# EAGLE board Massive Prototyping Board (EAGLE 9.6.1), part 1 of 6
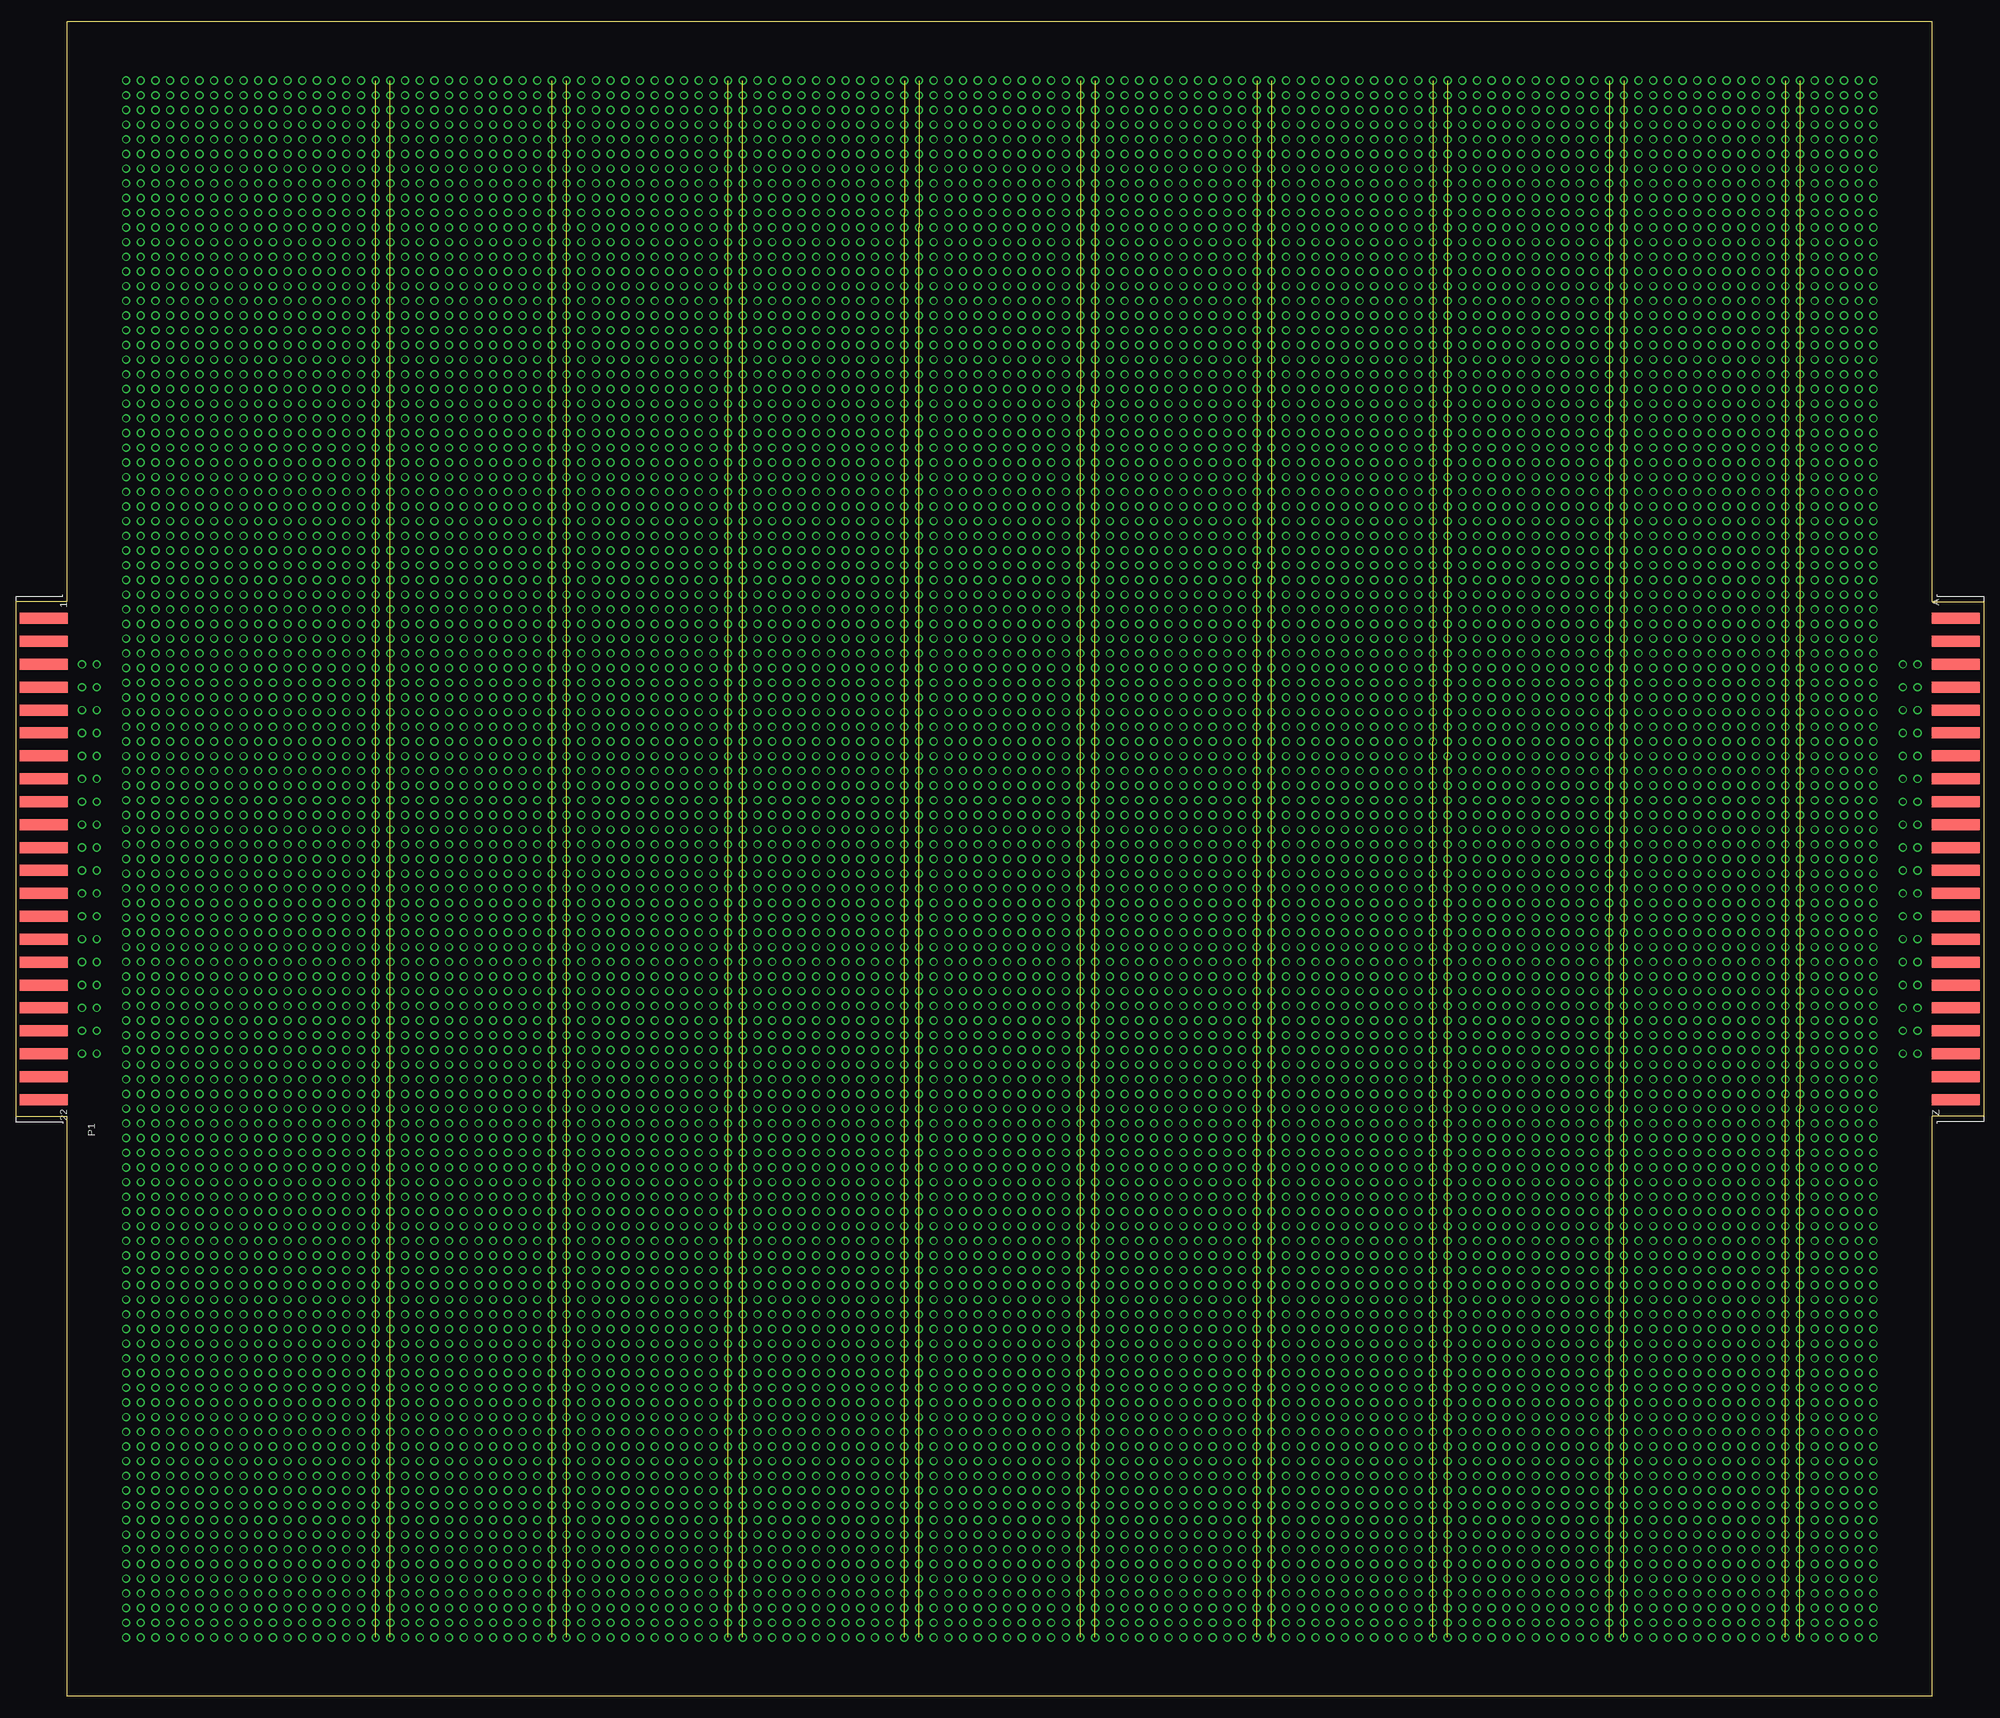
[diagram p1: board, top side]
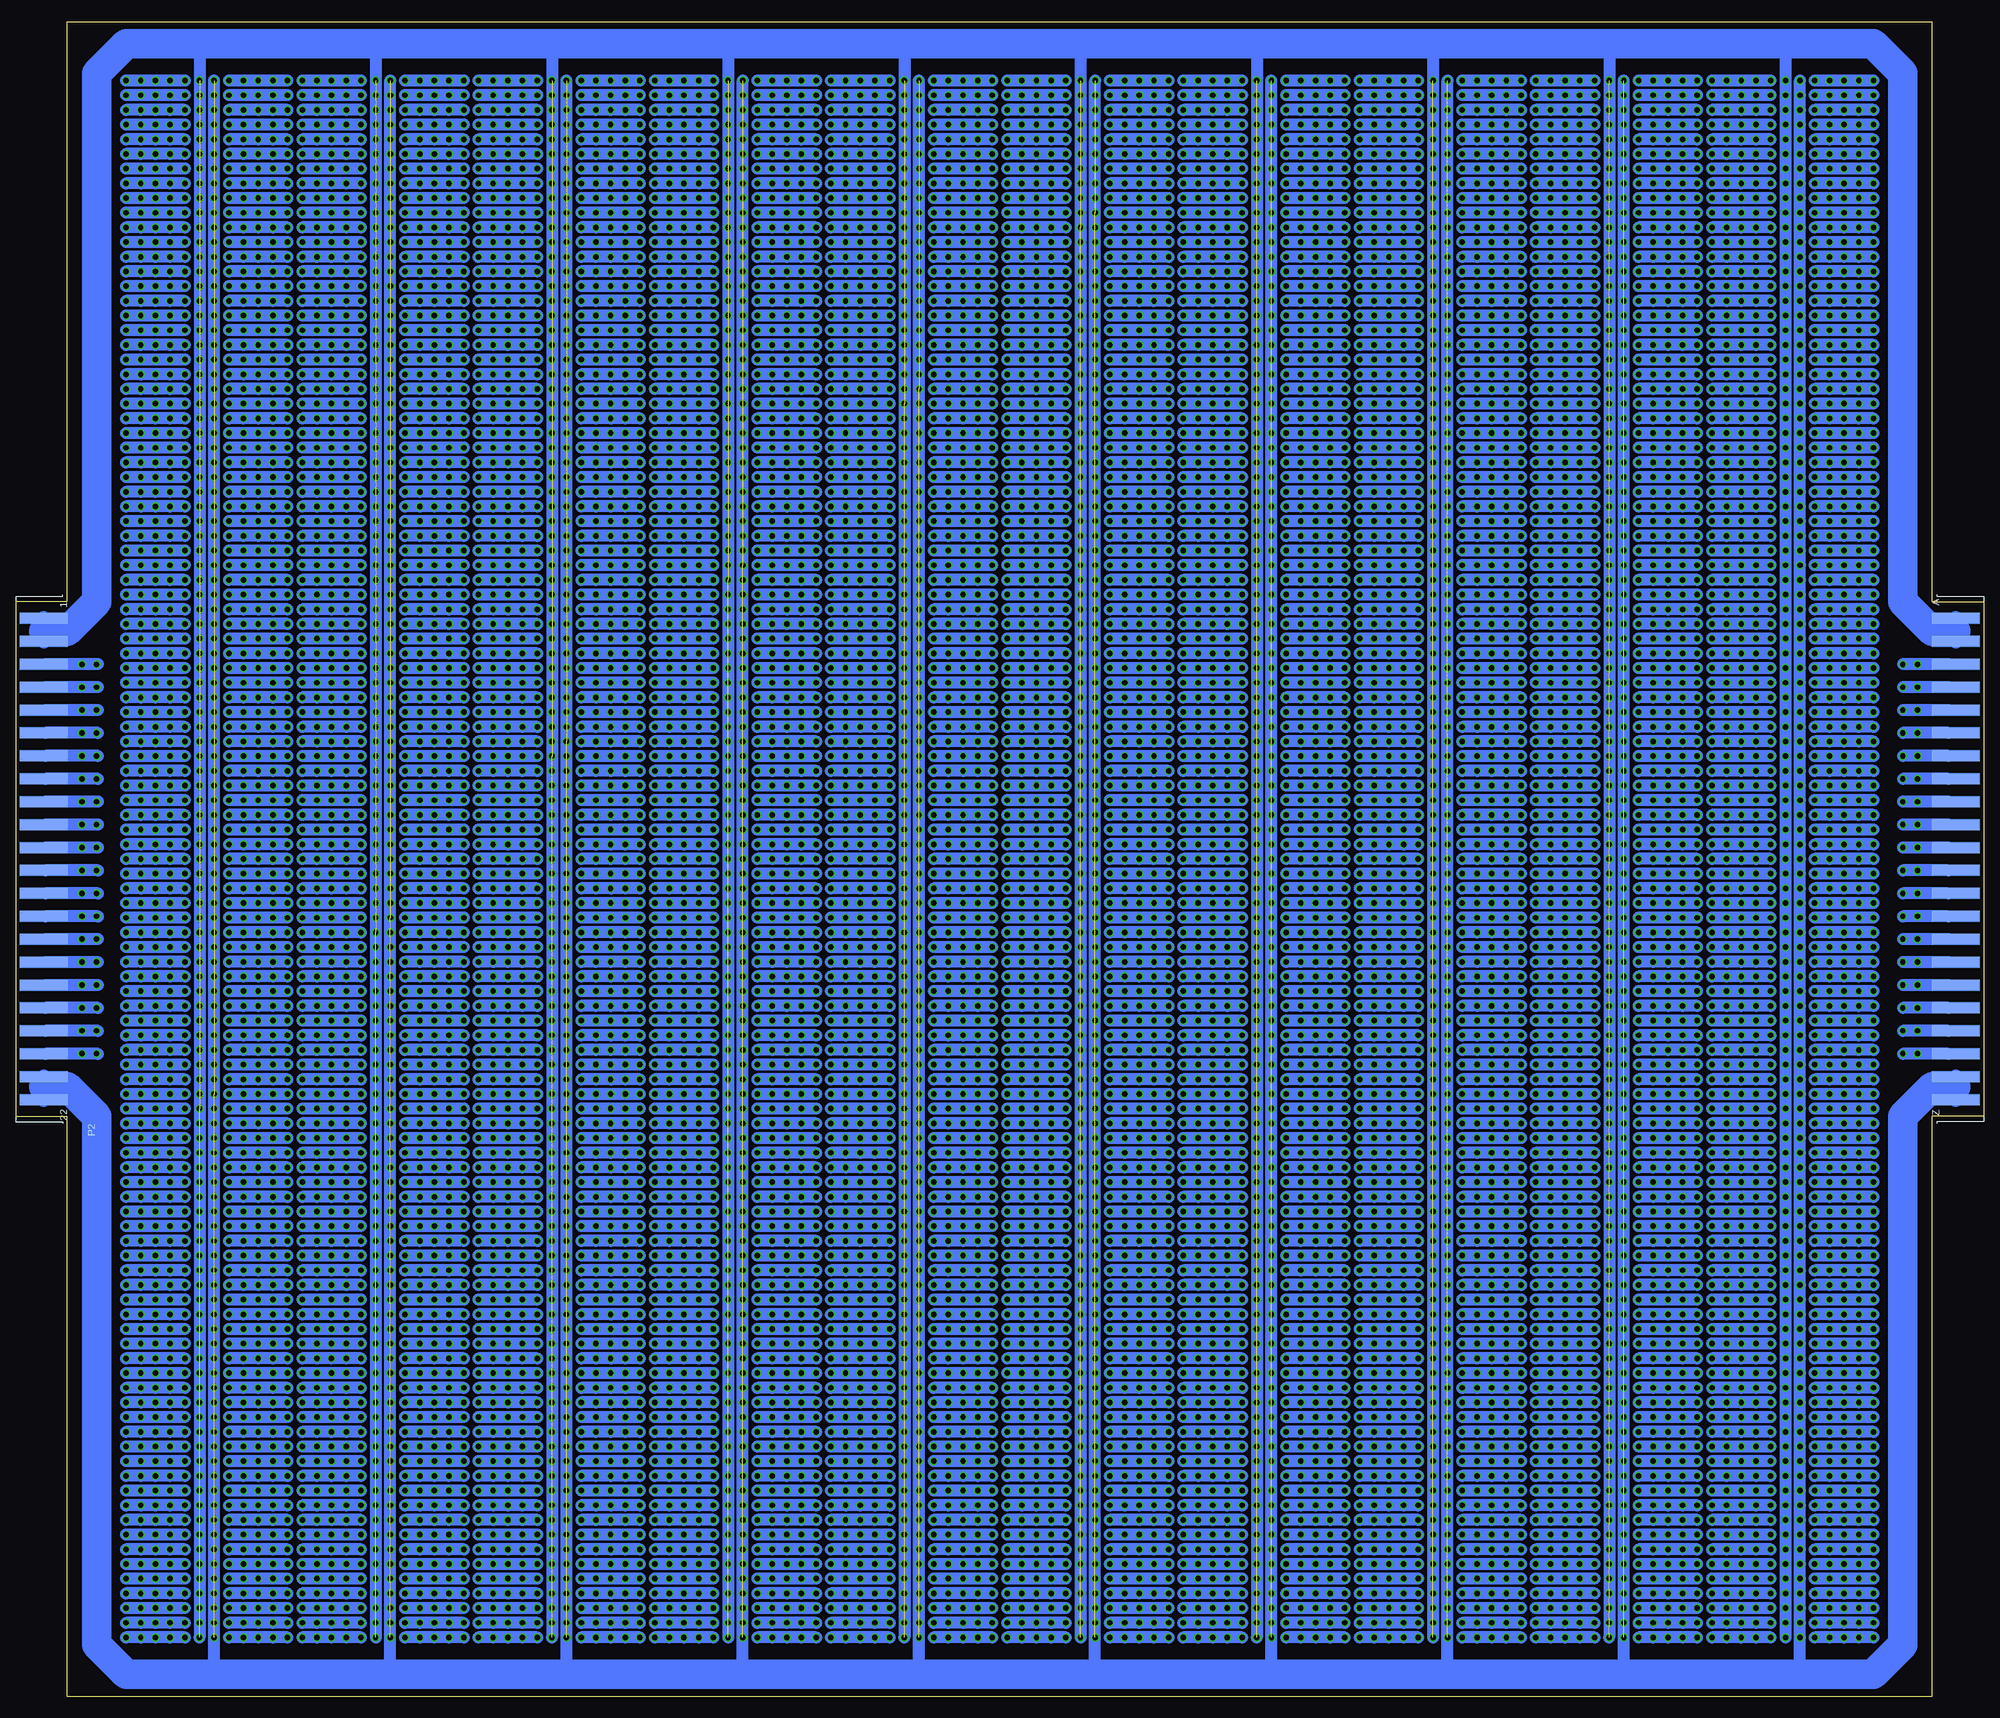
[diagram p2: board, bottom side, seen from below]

Size 340.36 x 289.56 mm. Coordinates in mm from the lower left corner, seen from the top.
Outline: 331.47,0 331.47,100.33 340.36,100.33 340.36,189.23 331.47,189.23 331.47,289.56 8.89,289.56 8.89,189.23 0,189.23 0,100.33 8.89,100.33 8.89,0 331.47,0
Copper layers (1*16): Top 0.035mm / dielectric 1.5mm / Bottom 0.035mm
Design rules "default": minimum track width 6mil, minimum drill 0.35mm, track to track 6mil, track to pad 6mil, pad to pad 6mil, via to via 6mil, smd to smd 6mil, copper to edge 40mil, drill to drill 6mil, minimum pad ring 10mil, minimum via ring 8mil, stop-mask expansion 4mil, vias tented up to drill 0mil, thermal gap 10mil

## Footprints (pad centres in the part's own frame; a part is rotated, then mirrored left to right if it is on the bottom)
44PINEDGE = smd 1.905 x 8.255: 1 -41.605,4.826; 2 -37.643,4.826; 3 -33.68,4.826; 4 -29.718,4.826; 5 -25.756,4.826; 6 -21.793,4.826; 7 -17.831,4.826; 8 -13.868,4.826; 9 -9.906,4.826; 10 -5.944,4.826; 11 -1.981,4.826; 12 1.981,4.826; 13 5.944,4.826; 14 9.906,4.826; 15 13.868,4.826; 16 17.831,4.826; 17 21.793,4.826; 18 25.756,4.826; 19 29.718,4.826; 20 33.68,4.826; 21 37.643,4.826; 22 41.605,4.826 | smd 1.905 x 8.255 bottom: A -41.605,4.826; B -37.643,4.826; C -33.68,4.826; D -29.718,4.826; E -25.756,4.826; F -21.793,4.826; H -17.831,4.826; J -13.868,4.826; K -9.906,4.826; L -5.944,4.826; M -1.981,4.826; N 1.981,4.826; P 5.944,4.826; R 9.906,4.826; S 13.868,4.826; T 17.831,4.826; U 21.793,4.826; V 25.756,4.826; W 29.718,4.826; X 33.68,4.826; Y 37.643,4.826; Z 41.605,4.826

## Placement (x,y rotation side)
P1  44PINEDGE  [44PINEDGE]  0,144.78 270 top
P2  44PINEDGE  [44PINEDGE]  340.36,144.78 270 bottom

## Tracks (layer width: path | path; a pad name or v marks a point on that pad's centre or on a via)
C1
  Bottom 2.032: 6.1,178.46 13.94,178.46
C2
  Bottom 2.032: 326.14,178.46 335.25,178.46
D1
  Bottom 2.032: 6.1,174.5 13.97,174.5
D2
  Bottom 2.032: 326.14,174.5 335.28,174.5
E1
  Bottom 2.032: 6.1,170.54 13.97,170.54
E2
  Bottom 2.032: 326.14,170.54 335.28,170.54
F1
  Bottom 2.032: 6.1,166.57 13.97,166.57
F2
  Bottom 2.032: 326.14,166.57 335.28,166.57
GND  (via drill 0.94)
  Bottom 2.032: 306.07,3.81 306.07,279.4 | 275.59,3.81 275.59,279.4 | 245.11,3.81 245.11,279.4 | 214.63,3.81 214.63,279.4 | 184.15,3.81 184.15,279.4 | 153.67,3.81 153.67,279.4 | 123.19,3.81 123.19,279.4 | 92.71,3.81 92.71,279.4 | 62.23,3.81 62.23,279.4 | 31.75,3.81 v31.75,10.16 v31.75,12.7 v31.75,15.24 v31.75,17.78 v31.75,20.32 v31.75,22.86 v31.75,25.4 v31.75,27.94 v31.75,30.48 v31.75,33.02 v31.75,35.56 v31.75,38.1 v31.75,40.64 v31.75,43.18 v31.75,45.72 v31.75,48.26 v31.75,50.8 v31.75,53.34 v31.75,55.88 v31.75,58.42 v31.75,60.96 v31.75,63.5 v31.75,66.04 v31.75,68.58 v31.75,71.12 v31.75,73.66 v31.75,76.2 v31.75,78.74 v31.75,81.28 v31.75,83.82 v31.75,86.36 v31.75,88.9 v31.75,91.44 v31.75,93.98 v31.75,96.52 v31.75,99.06 v31.75,101.6 v31.75,104.14 v31.75,106.68 v31.75,109.22 v31.75,111.76 v31.75,114.3 v31.75,116.84 v31.75,119.38 v31.75,121.92 v31.75,124.46 v31.75,127 v31.75,129.54 v31.75,132.08 v31.75,134.62 v31.75,137.16 v31.75,139.7 v31.75,142.24 v31.75,144.78 v31.75,147.32 v31.75,149.86 v31.75,152.4 v31.75,154.94 v31.75,157.48 v31.75,160.02 v31.75,162.56 v31.75,165.1 v31.75,167.64 v31.75,170.18 v31.75,172.72 v31.75,175.26 v31.75,177.8 v31.75,180.34 v31.75,182.88 v31.75,185.42 v31.75,187.96 v31.75,190.5 v31.75,193.04 v31.75,195.58 v31.75,198.12 v31.75,200.66 v31.75,203.2 v31.75,205.74 v31.75,208.28 v31.75,210.82 v31.75,213.36 v31.75,215.9 v31.75,218.44 v31.75,220.98 v31.75,223.52 v31.75,226.06 v31.75,228.6 v31.75,231.14 v31.75,233.68 v31.75,236.22 v31.75,238.76 v31.75,241.3 v31.75,243.84 v31.75,246.38 v31.75,248.92 v31.75,251.46 v31.75,254 v31.75,256.54 v31.75,259.08 v31.75,261.62 v31.75,264.16 v31.75,266.7 v31.75,269.24 v31.75,271.78 v31.75,274.32 v31.75,276.86 v31.75,279.4
  Bottom 2.54: P1.Y 4.83,105.41 P1.Z | P2.22 335.53,105.41 P2.21
  Bottom 5.08: 4.83,105.41 8.89,105.41 13.97,100.33 13.97,8.89 19.05,3.81 31.75,3.81 62.23,3.81 92.71,3.81 123.19,3.81 153.67,3.81 184.15,3.81 214.63,3.81 245.11,3.81 275.59,3.81 306.07,3.81 321.31,3.81 326.39,8.89 326.39,100.33 331.47,105.41 335.53,105.41
GND1  (via drill 0.94)  (106 unrouted)
  other vias: 62.23,10.16 62.23,12.7 62.23,15.24 62.23,17.78 62.23,20.32 62.23,22.86 62.23,25.4 62.23,27.94 62.23,30.48 62.23,33.02 62.23,35.56 62.23,38.1 62.23,40.64 62.23,43.18 62.23,45.72 62.23,48.26 62.23,50.8 62.23,53.34 62.23,55.88 62.23,58.42 62.23,63.5 62.23,60.96 62.23,66.04 62.23,68.58 62.23,71.12 62.23,73.66 62.23,76.2 62.23,78.74 62.23,83.82 62.23,81.28 62.23,86.36 62.23,88.9 62.23,91.44 62.23,93.98 62.23,96.52 62.23,99.06 62.23,101.6 62.23,104.14 62.23,106.68 62.23,109.22 62.23,111.76 62.23,114.3 62.23,116.84 62.23,119.38 62.23,121.92 62.23,124.46 62.23,127 62.23,129.54 62.23,132.08 62.23,134.62 62.23,137.16 62.23,139.7 62.23,142.24 62.23,144.78 62.23,147.32 62.23,149.86 62.23,152.4 62.23,154.94 62.23,157.48 62.23,160.02 62.23,162.56 62.23,165.1 62.23,167.64 62.23,170.18 62.23,172.72 62.23,175.26 62.23,177.8 62.23,180.34 62.23,185.42 62.23,182.88 62.23,187.96 62.23,190.5 62.23,193.04 62.23,195.58 62.23,198.12 62.23,200.66 62.23,203.2 62.23,205.74 62.23,208.28 62.23,210.82 62.23,213.36 62.23,215.9 62.23,218.44 62.23,220.98 62.23,223.52 62.23,226.06 62.23,228.6 62.23,231.14 62.23,233.68 62.23,236.22 62.23,238.76 62.23,241.3 62.23,243.84 62.23,246.38 62.23,248.92 62.23,251.46 62.23,254 62.23,256.54 62.23,259.08 62.23,261.62 62.23,264.16 62.23,266.7 62.23,269.24 62.23,271.78 62.23,274.32 62.23,276.86 62.23,279.4
GND2  (via drill 0.94)  (106 unrouted)
  other vias: 92.71,10.16 92.71,12.7 92.71,15.24 92.71,17.78 92.71,20.32 92.71,22.86 92.71,25.4 92.71,27.94 92.71,30.48 92.71,33.02 92.71,35.56 92.71,38.1 92.71,40.64 92.71,43.18 92.71,45.72 92.71,48.26 92.71,50.8 92.71,53.34 92.71,55.88 92.71,58.42 92.71,63.5 92.71,60.96 92.71,66.04 92.71,68.58 92.71,71.12 92.71,73.66 92.71,76.2 92.71,78.74 92.71,83.82 92.71,81.28 92.71,86.36 92.71,88.9 92.71,91.44 92.71,93.98 92.71,96.52 92.71,99.06 92.71,101.6 92.71,104.14 92.71,106.68 92.71,109.22 92.71,111.76 92.71,114.3 92.71,116.84 92.71,119.38 92.71,121.92 92.71,124.46 92.71,127 92.71,129.54 92.71,132.08 92.71,134.62 92.71,137.16 92.71,139.7 92.71,142.24 92.71,144.78 92.71,147.32 92.71,149.86 92.71,152.4 92.71,154.94 92.71,157.48 92.71,160.02 92.71,162.56 92.71,165.1 92.71,167.64 92.71,170.18 92.71,172.72 92.71,175.26 92.71,177.8 92.71,180.34 92.71,185.42 92.71,182.88 92.71,187.96 92.71,190.5 92.71,193.04 92.71,195.58 92.71,198.12 92.71,200.66 92.71,203.2 92.71,205.74 92.71,208.28 92.71,210.82 92.71,213.36 92.71,215.9 92.71,218.44 92.71,220.98 92.71,223.52 92.71,226.06 92.71,228.6 92.71,231.14 92.71,233.68 92.71,236.22 92.71,238.76 92.71,241.3 92.71,243.84 92.71,246.38 92.71,248.92 92.71,251.46 92.71,254 92.71,256.54 92.71,259.08 92.71,261.62 92.71,264.16 92.71,266.7 92.71,269.24 92.71,271.78 92.71,274.32 92.71,276.86 92.71,279.4
GND3  (via drill 0.94)  (106 unrouted)
  other vias: 123.19,10.16 123.19,12.7 123.19,15.24 123.19,17.78 123.19,20.32 123.19,22.86 123.19,25.4 123.19,27.94 123.19,30.48 123.19,33.02 123.19,35.56 123.19,38.1 123.19,40.64 123.19,43.18 123.19,45.72 123.19,48.26 123.19,50.8 123.19,53.34 123.19,55.88 123.19,58.42 123.19,63.5 123.19,60.96 123.19,66.04 123.19,68.58 123.19,71.12 123.19,73.66 123.19,76.2 123.19,78.74 123.19,83.82 123.19,81.28 123.19,86.36 123.19,88.9 123.19,91.44 123.19,93.98 123.19,96.52 123.19,99.06 123.19,101.6 123.19,104.14 123.19,106.68 123.19,109.22 123.19,111.76 123.19,114.3 123.19,116.84 123.19,119.38 123.19,121.92 123.19,124.46 123.19,127 123.19,129.54 123.19,132.08 123.19,134.62 123.19,137.16 123.19,139.7 123.19,142.24 123.19,144.78 123.19,147.32 123.19,149.86 123.19,152.4 123.19,154.94 123.19,157.48 123.19,160.02 123.19,162.56 123.19,165.1 123.19,167.64 123.19,170.18 123.19,172.72 123.19,175.26 123.19,177.8 123.19,180.34 123.19,185.42 123.19,182.88 123.19,187.96 123.19,190.5 123.19,193.04 123.19,195.58 123.19,198.12 123.19,200.66 123.19,203.2 123.19,205.74 123.19,208.28 123.19,210.82 123.19,213.36 123.19,215.9 123.19,218.44 123.19,220.98 123.19,223.52 123.19,226.06 123.19,228.6 123.19,231.14 123.19,233.68 123.19,236.22 123.19,238.76 123.19,241.3 123.19,243.84 123.19,246.38 123.19,248.92 123.19,251.46 123.19,254 123.19,256.54 123.19,259.08 123.19,261.62 123.19,264.16 123.19,266.7 123.19,269.24 123.19,271.78 123.19,274.32 123.19,276.86 123.19,279.4
GND4  (via drill 0.94)  (106 unrouted)
  other vias: 153.67,10.16 153.67,12.7 153.67,15.24 153.67,17.78 153.67,20.32 153.67,22.86 153.67,25.4 153.67,27.94 153.67,30.48 153.67,33.02 153.67,35.56 153.67,38.1 153.67,40.64 153.67,43.18 153.67,45.72 153.67,48.26 153.67,50.8 153.67,53.34 153.67,55.88 153.67,58.42 153.67,63.5 153.67,60.96 153.67,66.04 153.67,68.58 153.67,71.12 153.67,73.66 153.67,76.2 153.67,78.74 153.67,83.82 153.67,81.28 153.67,86.36 153.67,88.9 153.67,91.44 153.67,93.98 153.67,96.52 153.67,99.06 153.67,101.6 153.67,104.14 153.67,106.68 153.67,109.22 153.67,111.76 153.67,114.3 153.67,116.84 153.67,119.38 153.67,121.92 153.67,124.46 153.67,127 153.67,129.54 153.67,132.08 153.67,134.62 153.67,137.16 153.67,139.7 153.67,142.24 153.67,144.78 153.67,147.32 153.67,149.86 153.67,152.4 153.67,154.94 153.67,157.48 153.67,160.02 153.67,162.56 153.67,165.1 153.67,167.64 153.67,170.18 153.67,172.72 153.67,175.26 153.67,177.8 153.67,180.34 153.67,185.42 153.67,182.88 153.67,187.96 153.67,190.5 153.67,193.04 153.67,195.58 153.67,198.12 153.67,200.66 153.67,203.2 153.67,205.74 153.67,208.28 153.67,210.82 153.67,213.36 153.67,215.9 153.67,218.44 153.67,220.98 153.67,223.52 153.67,226.06 153.67,228.6 153.67,231.14 153.67,233.68 153.67,236.22 153.67,238.76 153.67,241.3 153.67,243.84 153.67,246.38 153.67,248.92 153.67,251.46 153.67,254 153.67,256.54 153.67,259.08 153.67,261.62 153.67,264.16 153.67,266.7 153.67,269.24 153.67,271.78 153.67,274.32 153.67,276.86 153.67,279.4
GND5  (via drill 0.94)  (106 unrouted)
  other vias: 184.15,10.16 184.15,12.7 184.15,15.24 184.15,17.78 184.15,20.32 184.15,22.86 184.15,25.4 184.15,27.94 184.15,30.48 184.15,33.02 184.15,35.56 184.15,38.1 184.15,40.64 184.15,43.18 184.15,45.72 184.15,48.26 184.15,50.8 184.15,53.34 184.15,55.88 184.15,58.42 184.15,63.5 184.15,60.96 184.15,66.04 184.15,68.58 184.15,71.12 184.15,73.66 184.15,76.2 184.15,78.74 184.15,83.82 184.15,81.28 184.15,86.36 184.15,88.9 184.15,91.44 184.15,93.98 184.15,96.52 184.15,99.06 184.15,101.6 184.15,104.14 184.15,106.68 184.15,109.22 184.15,111.76 184.15,114.3 184.15,116.84 184.15,119.38 184.15,121.92 184.15,124.46 184.15,127 184.15,129.54 184.15,132.08 184.15,134.62 184.15,137.16 184.15,139.7 184.15,142.24 184.15,144.78 184.15,147.32 184.15,149.86 184.15,152.4 184.15,154.94 184.15,157.48 184.15,160.02 184.15,162.56 184.15,165.1 184.15,167.64 184.15,170.18 184.15,172.72 184.15,175.26 184.15,177.8 184.15,180.34 184.15,185.42 184.15,182.88 184.15,187.96 184.15,190.5 184.15,193.04 184.15,195.58 184.15,198.12 184.15,200.66 184.15,203.2 184.15,205.74 184.15,208.28 184.15,210.82 184.15,213.36 184.15,215.9 184.15,218.44 184.15,220.98 184.15,223.52 184.15,226.06 184.15,228.6 184.15,231.14 184.15,233.68 184.15,236.22 184.15,238.76 184.15,241.3 184.15,243.84 184.15,246.38 184.15,248.92 184.15,251.46 184.15,254 184.15,256.54 184.15,259.08 184.15,261.62 184.15,264.16 184.15,266.7 184.15,269.24 184.15,271.78 184.15,274.32 184.15,276.86 184.15,279.4
GND6  (via drill 0.94)  (106 unrouted)
  other vias: 214.63,10.16 214.63,12.7 214.63,15.24 214.63,17.78 214.63,20.32 214.63,22.86 214.63,25.4 214.63,27.94 214.63,30.48 214.63,33.02 214.63,35.56 214.63,38.1 214.63,40.64 214.63,43.18 214.63,45.72 214.63,48.26 214.63,50.8 214.63,53.34 214.63,55.88 214.63,58.42 214.63,63.5 214.63,60.96 214.63,66.04 214.63,68.58 214.63,71.12 214.63,73.66 214.63,76.2 214.63,78.74 214.63,83.82 214.63,81.28 214.63,86.36 214.63,88.9 214.63,91.44 214.63,93.98 214.63,96.52 214.63,99.06 214.63,101.6 214.63,104.14 214.63,106.68 214.63,109.22 214.63,111.76 214.63,114.3 214.63,116.84 214.63,119.38 214.63,121.92 214.63,124.46 214.63,127 214.63,129.54 214.63,132.08 214.63,134.62 214.63,137.16 214.63,139.7 214.63,142.24 214.63,144.78 214.63,147.32 214.63,149.86 214.63,152.4 214.63,154.94 214.63,157.48 214.63,160.02 214.63,162.56 214.63,165.1 214.63,167.64 214.63,170.18 214.63,172.72 214.63,175.26 214.63,177.8 214.63,180.34 214.63,185.42 214.63,182.88 214.63,187.96 214.63,190.5 214.63,193.04 214.63,195.58 214.63,198.12 214.63,200.66 214.63,203.2 214.63,205.74 214.63,208.28 214.63,210.82 214.63,213.36 214.63,215.9 214.63,218.44 214.63,220.98 214.63,223.52 214.63,226.06 214.63,228.6 214.63,231.14 214.63,233.68 214.63,236.22 214.63,238.76 214.63,241.3 214.63,243.84 214.63,246.38 214.63,248.92 214.63,251.46 214.63,254 214.63,256.54 214.63,259.08 214.63,261.62 214.63,264.16 214.63,266.7 214.63,269.24 214.63,271.78 214.63,274.32 214.63,276.86 214.63,279.4
GND7  (via drill 0.94)  (106 unrouted)
  other vias: 245.11,10.16 245.11,12.7 245.11,15.24 245.11,17.78 245.11,20.32 245.11,22.86 245.11,25.4 245.11,27.94 245.11,30.48 245.11,33.02 245.11,35.56 245.11,38.1 245.11,40.64 245.11,43.18 245.11,45.72 245.11,48.26 245.11,50.8 245.11,53.34 245.11,55.88 245.11,58.42 245.11,63.5 245.11,60.96 245.11,66.04 245.11,68.58 245.11,71.12 245.11,73.66 245.11,76.2 245.11,78.74 245.11,83.82 245.11,81.28 245.11,86.36 245.11,88.9 245.11,91.44 245.11,93.98 245.11,96.52 245.11,99.06 245.11,101.6 245.11,104.14 245.11,106.68 245.11,109.22 245.11,111.76 245.11,114.3 245.11,116.84 245.11,119.38 245.11,121.92 245.11,124.46 245.11,127 245.11,129.54 245.11,132.08 245.11,134.62 245.11,137.16 245.11,139.7 245.11,142.24 245.11,144.78 245.11,147.32 245.11,149.86 245.11,152.4 245.11,154.94 245.11,157.48 245.11,160.02 245.11,162.56 245.11,165.1 245.11,167.64 245.11,170.18 245.11,172.72 245.11,175.26 245.11,177.8 245.11,180.34 245.11,185.42 245.11,182.88 245.11,187.96 245.11,190.5 245.11,193.04 245.11,195.58 245.11,198.12 245.11,200.66 245.11,203.2 245.11,205.74 245.11,208.28 245.11,210.82 245.11,213.36 245.11,215.9 245.11,218.44 245.11,220.98 245.11,223.52 245.11,226.06 245.11,228.6 245.11,231.14 245.11,233.68 245.11,236.22 245.11,238.76 245.11,241.3 245.11,243.84 245.11,246.38 245.11,248.92 245.11,251.46 245.11,254 245.11,256.54 245.11,259.08 245.11,261.62 245.11,264.16 245.11,266.7 245.11,269.24 245.11,271.78 245.11,274.32 245.11,276.86 245.11,279.4
GND8  (via drill 0.94)  (106 unrouted)
  other vias: 275.59,10.16 275.59,12.7 275.59,15.24 275.59,17.78 275.59,20.32 275.59,22.86 275.59,25.4 275.59,27.94 275.59,30.48 275.59,33.02 275.59,35.56 275.59,38.1 275.59,40.64 275.59,43.18 275.59,45.72 275.59,48.26 275.59,50.8 275.59,53.34 275.59,55.88 275.59,58.42 275.59,63.5 275.59,60.96 275.59,66.04 275.59,68.58 275.59,71.12 275.59,73.66 275.59,76.2 275.59,78.74 275.59,83.82 275.59,81.28 275.59,86.36 275.59,88.9 275.59,91.44 275.59,93.98 275.59,96.52 275.59,99.06 275.59,101.6 275.59,104.14 275.59,106.68 275.59,109.22 275.59,111.76 275.59,114.3 275.59,116.84 275.59,119.38 275.59,121.92 275.59,124.46 275.59,127 275.59,129.54 275.59,132.08 275.59,134.62 275.59,137.16 275.59,139.7 275.59,142.24 275.59,144.78 275.59,147.32 275.59,149.86 275.59,152.4 275.59,154.94 275.59,157.48 275.59,160.02 275.59,162.56 275.59,165.1 275.59,167.64 275.59,170.18 275.59,172.72 275.59,175.26 275.59,177.8 275.59,180.34 275.59,185.42 275.59,182.88 275.59,187.96 275.59,190.5 275.59,193.04 275.59,195.58 275.59,198.12 275.59,200.66 275.59,203.2 275.59,205.74 275.59,208.28 275.59,210.82 275.59,213.36 275.59,215.9 275.59,218.44 275.59,220.98 275.59,223.52 275.59,226.06 275.59,228.6 275.59,231.14 275.59,233.68 275.59,236.22 275.59,238.76 275.59,241.3 275.59,243.84 275.59,246.38 275.59,248.92 275.59,251.46 275.59,254 275.59,256.54 275.59,259.08 275.59,261.62 275.59,264.16 275.59,266.7 275.59,269.24 275.59,271.78 275.59,274.32 275.59,276.86 275.59,279.4
GND9  (via drill 0.94)  (106 unrouted)
  other vias: 306.07,10.16 306.07,12.7 306.07,15.24 306.07,17.78 306.07,20.32 306.07,22.86 306.07,25.4 306.07,27.94 306.07,30.48 306.07,33.02 306.07,35.56 306.07,38.1 306.07,40.64 306.07,43.18 306.07,45.72 306.07,48.26 306.07,50.8 306.07,53.34 306.07,55.88 306.07,58.42 306.07,63.5 306.07,60.96 306.07,66.04 306.07,68.58 306.07,71.12 306.07,73.66 306.07,76.2 306.07,78.74 306.07,83.82 306.07,81.28 306.07,86.36 306.07,88.9 306.07,91.44 306.07,93.98 306.07,96.52 306.07,99.06 306.07,101.6 306.07,104.14 306.07,106.68 306.07,109.22 306.07,111.76 306.07,114.3 306.07,116.84 306.07,119.38 306.07,121.92 306.07,124.46 306.07,127 306.07,129.54 306.07,132.08 306.07,134.62 306.07,137.16 306.07,139.7 306.07,142.24 306.07,144.78 306.07,147.32 306.07,149.86 306.07,152.4 306.07,154.94 306.07,157.48 306.07,160.02 306.07,162.56 306.07,165.1 306.07,167.64 306.07,170.18 306.07,172.72 306.07,175.26 306.07,177.8 306.07,180.34 306.07,185.42 306.07,182.88 306.07,187.96 306.07,190.5 306.07,193.04 306.07,195.58 306.07,198.12 306.07,200.66 306.07,203.2 306.07,205.74 306.07,208.28 306.07,210.82 306.07,213.36 306.07,215.9 306.07,218.44 306.07,220.98 306.07,223.52 306.07,226.06 306.07,228.6 306.07,231.14 306.07,233.68 306.07,236.22 306.07,238.76 306.07,241.3 306.07,243.84 306.07,246.38 306.07,248.92 306.07,251.46 306.07,254 306.07,256.54 306.07,259.08 306.07,261.62 306.07,264.16 306.07,266.7 306.07,269.24 306.07,271.78 306.07,274.32 306.07,276.86 306.07,279.4
H1
  Bottom 2.032: 6.1,162.61 13.97,162.61
H2
  Bottom 2.032: 326.14,162.61 335.28,162.61
J1
  Bottom 2.032: 6.1,158.65 13.97,158.65
J2
  Bottom 2.032: 326.14,158.65 335.28,158.65
K1
  Bottom 2.032: 6.1,154.69 13.97,154.69
K2
  Bottom 2.032: 326.14,154.69 335.28,154.69
L1
  Bottom 2.032: 6.1,150.72 13.97,150.72
L2
  Bottom 2.032: 326.14,150.72 335.28,150.72
M1
  Bottom 2.032: 6.1,146.76 13.97,146.76
M2
  Bottom 2.032: 326.14,146.76 335.28,146.76
N1
  Bottom 2.032: 6.1,142.8 13.97,142.8
N2
  Bottom 2.032: 326.14,142.8 335.28,142.8
N$1  (via drill 0.94)
  Bottom 2.032: v36.83,12.7 v39.37,12.7 v41.91,12.7 v44.45,12.7 v46.99,12.7
N$2  (via drill 0.94)
  Bottom 2.032: v36.83,15.24 v39.37,15.24 v41.91,15.24 v44.45,15.24 v46.99,15.24
N$3  (via drill 0.94)
  Bottom 2.032: v36.83,17.78 v39.37,17.78 v41.91,17.78 v44.45,17.78 v46.99,17.78
N$4  (via drill 0.94)
  Bottom 2.032: v36.83,20.32 v39.37,20.32 v41.91,20.32 v44.45,20.32 v46.99,20.32
N$5  (via drill 0.94)
  Bottom 2.032: v36.83,22.86 v39.37,22.86 v41.91,22.86 v44.45,22.86 v46.99,22.86
N$6  (via drill 0.94)
  Bottom 2.032: v36.83,25.4 v39.37,25.4 v41.91,25.4 v44.45,25.4 v46.99,25.4
N$7  (via drill 0.94)
  Bottom 2.032: v36.83,27.94 v39.37,27.94 v41.91,27.94 v44.45,27.94 v46.99,27.94
N$8  (via drill 0.94)
  Bottom 2.032: v36.83,30.48 v39.37,30.48 v41.91,30.48 v44.45,30.48 v46.99,30.48
N$9  (via drill 0.94)
  Bottom 2.032: v36.83,33.02 v39.37,33.02 v41.91,33.02 v44.45,33.02 v46.99,33.02
N$10  (via drill 0.94)
  Bottom 2.032: v36.83,35.56 v39.37,35.56 v41.91,35.56 v44.45,35.56 v46.99,35.56
N$11  (via drill 0.94)
  Bottom 2.032: v36.83,38.1 v39.37,38.1 v41.91,38.1 v44.45,38.1 v46.99,38.1
N$12  (via drill 0.94)
  Bottom 2.032: v36.83,40.64 v39.37,40.64 v41.91,40.64 v44.45,40.64 v46.99,40.64
N$13  (via drill 0.94)
  Bottom 2.032: v36.83,43.18 v39.37,43.18 v41.91,43.18 v44.45,43.18 v46.99,43.18
N$14  (via drill 0.94)
  Bottom 2.032: v36.83,45.72 v39.37,45.72 v41.91,45.72 v44.45,45.72 v46.99,45.72
N$15  (via drill 0.94)
  Bottom 2.032: v36.83,48.26 v39.37,48.26 v41.91,48.26 v44.45,48.26 v46.99,48.26
N$16  (via drill 0.94)
  Bottom 2.032: v36.83,50.8 v39.37,50.8 v41.91,50.8 v44.45,50.8 v46.99,50.8
N$17  (via drill 0.94)
  Bottom 2.032: v36.83,53.34 v39.37,53.34 v41.91,53.34 v44.45,53.34 v46.99,53.34
N$18  (via drill 0.94)
  Bottom 2.032: v36.83,55.88 v39.37,55.88 v41.91,55.88 v44.45,55.88 v46.99,55.88
N$19  (via drill 0.94)
  Bottom 2.032: v36.83,58.42 v39.37,58.42 v41.91,58.42 v44.45,58.42 v46.99,58.42
N$20  (via drill 0.94)
  Bottom 2.032: v36.83,60.96 v39.37,60.96 v41.91,60.96 v44.45,60.96 v46.99,60.96
N$21  (via drill 0.94)
  Bottom 2.032: v36.83,63.5 v39.37,63.5 v41.91,63.5 v44.45,63.5 v46.99,63.5
N$22  (via drill 0.94)
  Bottom 2.032: v36.83,66.04 v39.37,66.04 v41.91,66.04 v44.45,66.04 v46.99,66.04
N$23  (via drill 0.94)
  Bottom 2.032: v36.83,68.58 v39.37,68.58 v41.91,68.58 v44.45,68.58 v46.99,68.58
N$24  (via drill 0.94)
  Bottom 2.032: v36.83,71.12 v39.37,71.12 v41.91,71.12 v44.45,71.12 v46.99,71.12
N$25  (via drill 0.94)
  Bottom 2.032: v36.83,73.66 v39.37,73.66 v41.91,73.66 v44.45,73.66 v46.99,73.66
N$26  (via drill 0.94)
  Bottom 2.032: v36.83,76.2 v39.37,76.2 v41.91,76.2 v44.45,76.2 v46.99,76.2
N$27  (via drill 0.94)
  Bottom 2.032: v36.83,78.74 v39.37,78.74 v41.91,78.74 v44.45,78.74 v46.99,78.74
N$28  (via drill 0.94)
  Bottom 2.032: v36.83,81.28 v39.37,81.28 v41.91,81.28 v44.45,81.28 v46.99,81.28
N$29  (via drill 0.94)
  Bottom 2.032: v36.83,83.82 v39.37,83.82 v41.91,83.82 v44.45,83.82 v46.99,83.82
N$30  (via drill 0.94)
  Bottom 2.032: v36.83,86.36 v39.37,86.36 v41.91,86.36 v44.45,86.36 v46.99,86.36
N$31  (via drill 0.94)
  Bottom 2.032: v36.83,88.9 v39.37,88.9 v41.91,88.9 v44.45,88.9 v46.99,88.9
N$32  (via drill 0.94)
  Bottom 2.032: v36.83,91.44 v39.37,91.44 v41.91,91.44 v44.45,91.44 v46.99,91.44
N$33  (via drill 0.94)
  Bottom 2.032: v36.83,93.98 v39.37,93.98 v41.91,93.98 v44.45,93.98 v46.99,93.98
N$34  (via drill 0.94)
  Bottom 2.032: v36.83,96.52 v39.37,96.52 v41.91,96.52 v44.45,96.52 v46.99,96.52
N$35  (via drill 0.94)
  Bottom 2.032: v36.83,99.06 v39.37,99.06 v41.91,99.06 v44.45,99.06 v46.99,99.06
N$36  (via drill 0.94)
  Bottom 2.032: v36.83,101.6 v39.37,101.6 v41.91,101.6 v44.45,101.6 v46.99,101.6
N$37  (via drill 0.94)
  Bottom 2.032: v36.83,104.14 v39.37,104.14 v41.91,104.14 v44.45,104.14 v46.99,104.14
N$38  (via drill 0.94)
  Bottom 2.032: v36.83,106.68 v39.37,106.68 v41.91,106.68 v44.45,106.68 v46.99,106.68
N$39  (via drill 0.94)
  Bottom 2.032: v36.83,109.22 v39.37,109.22 v41.91,109.22 v44.45,109.22 v46.99,109.22
N$40  (via drill 0.94)
  Bottom 2.032: v36.83,111.76 v39.37,111.76 v41.91,111.76 v44.45,111.76 v46.99,111.76
N$41  (via drill 0.94)
  Bottom 2.032: v36.83,114.3 v39.37,114.3 v41.91,114.3 v44.45,114.3 v46.99,114.3
N$42  (via drill 0.94)
  Bottom 2.032: v36.83,116.84 v39.37,116.84 v41.91,116.84 v44.45,116.84 v46.99,116.84
N$43  (via drill 0.94)
  Bottom 2.032: v36.83,119.38 v39.37,119.38 v41.91,119.38 v44.45,119.38 v46.99,119.38
N$44  (via drill 0.94)
  Bottom 2.032: v36.83,121.92 v39.37,121.92 v41.91,121.92 v44.45,121.92 v46.99,121.92
N$45  (via drill 0.94)
  Bottom 2.032: v36.83,124.46 v39.37,124.46 v41.91,124.46 v44.45,124.46 v46.99,124.46
N$46  (via drill 0.94)
  Bottom 2.032: v36.83,127 v39.37,127 v41.91,127 v44.45,127 v46.99,127
N$47  (via drill 0.94)
  Bottom 2.032: v36.83,129.54 v39.37,129.54 v41.91,129.54 v44.45,129.54 v46.99,129.54
N$48  (via drill 0.94)
  Bottom 2.032: v36.83,132.08 v39.37,132.08 v41.91,132.08 v44.45,132.08 v46.99,132.08
N$49  (via drill 0.94)
  Bottom 2.032: v36.83,134.62 v39.37,134.62 v41.91,134.62 v44.45,134.62 v46.99,134.62
N$50  (via drill 0.94)
  Bottom 2.032: v36.83,137.16 v39.37,137.16 v41.91,137.16 v44.45,137.16 v46.99,137.16
N$51  (via drill 0.94)
  Bottom 2.032: v36.83,139.7 v39.37,139.7 v41.91,139.7 v44.45,139.7 v46.99,139.7
N$52  (via drill 0.94)
  Bottom 2.032: v36.83,142.24 v39.37,142.24 v41.91,142.24 v44.45,142.24 v46.99,142.24
N$53  (via drill 0.94)
  Bottom 2.032: v36.83,144.78 v39.37,144.78 v41.91,144.78 v44.45,144.78 v46.99,144.78
N$54  (via drill 0.94)
  Bottom 2.032: v36.83,147.32 v39.37,147.32 v41.91,147.32 v44.45,147.32 v46.99,147.32
N$55  (via drill 0.94)
  Bottom 2.032: v36.83,149.86 v39.37,149.86 v41.91,149.86 v44.45,149.86 v46.99,149.86
N$56  (via drill 0.94)
  Bottom 2.032: v36.83,152.4 v39.37,152.4 v41.91,152.4 v44.45,152.4 v46.99,152.4
N$57  (via drill 0.94)
  Bottom 2.032: v36.83,154.94 v39.37,154.94 v41.91,154.94 v44.45,154.94 v46.99,154.94
N$58  (via drill 0.94)
  Bottom 2.032: v36.83,157.48 v39.37,157.48 v41.91,157.48 v44.45,157.48 v46.99,157.48
N$59  (via drill 0.94)
  Bottom 2.032: v36.83,160.02 v39.37,160.02 v41.91,160.02 v44.45,160.02 v46.99,160.02
N$60  (via drill 0.94)
  Bottom 2.032: v36.83,162.56 v39.37,162.56 v41.91,162.56 v44.45,162.56 v46.99,162.56
N$61  (via drill 0.94)
  Bottom 2.032: v36.83,165.1 v39.37,165.1 v41.91,165.1 v44.45,165.1 v46.99,165.1
N$62  (via drill 0.94)
  Bottom 2.032: v36.83,167.64 v39.37,167.64 v41.91,167.64 v44.45,167.64 v46.99,167.64
N$63  (via drill 0.94)
  Bottom 2.032: v36.83,170.18 v39.37,170.18 v41.91,170.18 v44.45,170.18 v46.99,170.18
N$64  (via drill 0.94)
  Bottom 2.032: v36.83,172.72 v39.37,172.72 v41.91,172.72 v44.45,172.72 v46.99,172.72
N$65  (via drill 0.94)
  Bottom 2.032: v36.83,175.26 v39.37,175.26 v41.91,175.26 v44.45,175.26 v46.99,175.26
N$66  (via drill 0.94)
  Bottom 2.032: v36.83,177.8 v39.37,177.8 v41.91,177.8 v44.45,177.8 v46.99,177.8
N$67  (via drill 0.94)
  Bottom 2.032: v36.83,180.34 v39.37,180.34 v41.91,180.34 v44.45,180.34 v46.99,180.34
N$68  (via drill 0.94)
  Bottom 2.032: v36.83,182.88 v39.37,182.88 v41.91,182.88 v44.45,182.88 v46.99,182.88
N$69  (via drill 0.94)
  Bottom 2.032: v36.83,185.42 v39.37,185.42 v41.91,185.42 v44.45,185.42 v46.99,185.42
N$70  (via drill 0.94)
  Bottom 2.032: v36.83,187.96 v39.37,187.96 v41.91,187.96 v44.45,187.96 v46.99,187.96
N$71  (via drill 0.94)
  Bottom 2.032: v36.83,190.5 v39.37,190.5 v41.91,190.5 v44.45,190.5 v46.99,190.5
N$72  (via drill 0.94)
  Bottom 2.032: v36.83,193.04 v39.37,193.04 v41.91,193.04 v44.45,193.04 v46.99,193.04
N$73  (via drill 0.94)
  Bottom 2.032: v36.83,195.58 v39.37,195.58 v41.91,195.58 v44.45,195.58 v46.99,195.58
N$74  (via drill 0.94)
  Bottom 2.032: v49.53,12.7 v52.07,12.7 v54.61,12.7 v57.15,12.7 v59.69,12.7
N$75  (via drill 0.94)
  Bottom 2.032: v49.53,15.24 v52.07,15.24 v54.61,15.24 v57.15,15.24 v59.69,15.24
N$76  (via drill 0.94)
  Bottom 2.032: v49.53,17.78 v52.07,17.78 v54.61,17.78 v57.15,17.78 v59.69,17.78
N$77  (via drill 0.94)
  Bottom 2.032: v49.53,20.32 v52.07,20.32 v54.61,20.32 v57.15,20.32 v59.69,20.32
N$78  (via drill 0.94)
  Bottom 2.032: v49.53,22.86 v52.07,22.86 v54.61,22.86 v57.15,22.86 v59.69,22.86
N$79  (via drill 0.94)
  Bottom 2.032: v49.53,25.4 v52.07,25.4 v54.61,25.4 v57.15,25.4 v59.69,25.4
N$80  (via drill 0.94)
  Bottom 2.032: v49.53,27.94 v52.07,27.94 v54.61,27.94 v57.15,27.94 v59.69,27.94
N$81  (via drill 0.94)
  Bottom 2.032: v49.53,30.48 v52.07,30.48 v54.61,30.48 v57.15,30.48 v59.69,30.48
N$82  (via drill 0.94)
  Bottom 2.032: v49.53,33.02 v52.07,33.02 v54.61,33.02 v57.15,33.02 v59.69,33.02
N$83  (via drill 0.94)
  Bottom 2.032: v49.53,35.56 v52.07,35.56 v54.61,35.56 v57.15,35.56 v59.69,35.56
N$84  (via drill 0.94)
  Bottom 2.032: v49.53,38.1 v52.07,38.1 v54.61,38.1 v57.15,38.1 v59.69,38.1
N$85  (via drill 0.94)
  Bottom 2.032: v49.53,40.64 v52.07,40.64 v54.61,40.64 v57.15,40.64 v59.69,40.64
N$86  (via drill 0.94)
  Bottom 2.032: v49.53,43.18 v52.07,43.18 v54.61,43.18 v57.15,43.18 v59.69,43.18
N$87  (via drill 0.94)
  Bottom 2.032: v49.53,45.72 v52.07,45.72 v54.61,45.72 v57.15,45.72 v59.69,45.72
N$88  (via drill 0.94)
  Bottom 2.032: v49.53,48.26 v52.07,48.26 v54.61,48.26 v57.15,48.26 v59.69,48.26
N$89  (via drill 0.94)
  Bottom 2.032: v49.53,50.8 v52.07,50.8 v54.61,50.8 v57.15,50.8 v59.69,50.8
N$90  (via drill 0.94)
  Bottom 2.032: v49.53,53.34 v52.07,53.34 v54.61,53.34 v57.15,53.34 v59.69,53.34
N$91  (via drill 0.94)
  Bottom 2.032: v49.53,55.88 v52.07,55.88 v54.61,55.88 v57.15,55.88 v59.69,55.88
N$92  (via drill 0.94)
  Bottom 2.032: v49.53,58.42 v52.07,58.42 v54.61,58.42 v57.15,58.42 v59.69,58.42
N$93  (via drill 0.94)
  Bottom 2.032: v49.53,60.96 v52.07,60.96 v54.61,60.96 v57.15,60.96 v59.69,60.96
N$94  (via drill 0.94)
  Bottom 2.032: v49.53,63.5 v52.07,63.5 v54.61,63.5 v57.15,63.5 v59.69,63.5
N$95  (via drill 0.94)
  Bottom 2.032: v49.53,66.04 v52.07,66.04 v54.61,66.04 v57.15,66.04 v59.69,66.04
N$96  (via drill 0.94)
  Bottom 2.032: v49.53,68.58 v52.07,68.58 v54.61,68.58 v57.15,68.58 v59.69,68.58
N$97  (via drill 0.94)
  Bottom 2.032: v49.53,71.12 v52.07,71.12 v54.61,71.12 v57.15,71.12 v59.69,71.12
N$98  (via drill 0.94)
  Bottom 2.032: v49.53,73.66 v52.07,73.66 v54.61,73.66 v57.15,73.66 v59.69,73.66
N$99  (via drill 0.94)
  Bottom 2.032: v49.53,76.2 v52.07,76.2 v54.61,76.2 v57.15,76.2 v59.69,76.2
N$100  (via drill 0.94)
  Bottom 2.032: v49.53,78.74 v52.07,78.74 v54.61,78.74 v57.15,78.74 v59.69,78.74
N$101  (via drill 0.94)
  Bottom 2.032: v49.53,81.28 v52.07,81.28 v54.61,81.28 v57.15,81.28 v59.69,81.28
N$102  (via drill 0.94)
  Bottom 2.032: v49.53,83.82 v52.07,83.82 v54.61,83.82 v57.15,83.82 v59.69,83.82
N$103  (via drill 0.94)
  Bottom 2.032: v49.53,86.36 v52.07,86.36 v54.61,86.36 v57.15,86.36 v59.69,86.36
N$104  (via drill 0.94)
  Bottom 2.032: v49.53,88.9 v52.07,88.9 v54.61,88.9 v57.15,88.9 v59.69,88.9
N$105  (via drill 0.94)
  Bottom 2.032: v49.53,91.44 v52.07,91.44 v54.61,91.44 v57.15,91.44 v59.69,91.44
N$106  (via drill 0.94)
  Bottom 2.032: v49.53,93.98 v52.07,93.98 v54.61,93.98 v57.15,93.98 v59.69,93.98
N$107  (via drill 0.94)
  Bottom 2.032: v49.53,96.52 v52.07,96.52 v54.61,96.52 v57.15,96.52 v59.69,96.52
N$108  (via drill 0.94)
  Bottom 2.032: v49.53,99.06 v52.07,99.06 v54.61,99.06 v57.15,99.06 v59.69,99.06
N$109  (via drill 0.94)
  Bottom 2.032: v49.53,101.6 v52.07,101.6 v54.61,101.6 v57.15,101.6 v59.69,101.6
N$110  (via drill 0.94)
  Bottom 2.032: v49.53,104.14 v52.07,104.14 v54.61,104.14 v57.15,104.14 v59.69,104.14
N$111  (via drill 0.94)
  Bottom 2.032: v49.53,106.68 v52.07,106.68 v54.61,106.68 v57.15,106.68 v59.69,106.68
N$112  (via drill 0.94)
  Bottom 2.032: v49.53,109.22 v52.07,109.22 v54.61,109.22 v57.15,109.22 v59.69,109.22
N$113  (via drill 0.94)
  Bottom 2.032: v49.53,111.76 v52.07,111.76 v54.61,111.76 v57.15,111.76 v59.69,111.76
N$114  (via drill 0.94)
  Bottom 2.032: v49.53,114.3 v52.07,114.3 v54.61,114.3 v57.15,114.3 v59.69,114.3
N$115  (via drill 0.94)
  Bottom 2.032: v49.53,116.84 v52.07,116.84 v54.61,116.84 v57.15,116.84 v59.69,116.84
N$116  (via drill 0.94)
  Bottom 2.032: v49.53,119.38 v52.07,119.38 v54.61,119.38 v57.15,119.38 v59.69,119.38
N$117  (via drill 0.94)
  Bottom 2.032: v49.53,121.92 v52.07,121.92 v54.61,121.92 v57.15,121.92 v59.69,121.92
N$118  (via drill 0.94)
  Bottom 2.032: v49.53,124.46 v52.07,124.46 v54.61,124.46 v57.15,124.46 v59.69,124.46
N$119  (via drill 0.94)
  Bottom 2.032: v49.53,127 v52.07,127 v54.61,127 v57.15,127 v59.69,127
N$120  (via drill 0.94)
  Bottom 2.032: v49.53,129.54 v52.07,129.54 v54.61,129.54 v57.15,129.54 v59.69,129.54
N$121  (via drill 0.94)
  Bottom 2.032: v49.53,132.08 v52.07,132.08 v54.61,132.08 v57.15,132.08 v59.69,132.08
N$122  (via drill 0.94)
  Bottom 2.032: v49.53,134.62 v52.07,134.62 v54.61,134.62 v57.15,134.62 v59.69,134.62
N$123  (via drill 0.94)
  Bottom 2.032: v49.53,137.16 v52.07,137.16 v54.61,137.16 v57.15,137.16 v59.69,137.16
N$124  (via drill 0.94)
  Bottom 2.032: v49.53,139.7 v52.07,139.7 v54.61,139.7 v57.15,139.7 v59.69,139.7
N$125  (via drill 0.94)
  Bottom 2.032: v49.53,142.24 v52.07,142.24 v54.61,142.24 v57.15,142.24 v59.69,142.24
N$126  (via drill 0.94)
  Bottom 2.032: v49.53,144.78 v52.07,144.78 v54.61,144.78 v57.15,144.78 v59.69,144.78
N$127  (via drill 0.94)
  Bottom 2.032: v49.53,147.32 v52.07,147.32 v54.61,147.32 v57.15,147.32 v59.69,147.32
N$128  (via drill 0.94)
  Bottom 2.032: v49.53,149.86 v52.07,149.86 v54.61,149.86 v57.15,149.86 v59.69,149.86
N$129  (via drill 0.94)
  Bottom 2.032: v49.53,152.4 v52.07,152.4 v54.61,152.4 v57.15,152.4 v59.69,152.4
N$130  (via drill 0.94)
  Bottom 2.032: v49.53,154.94 v52.07,154.94 v54.61,154.94 v57.15,154.94 v59.69,154.94
N$131  (via drill 0.94)
  Bottom 2.032: v49.53,157.48 v52.07,157.48 v54.61,157.48 v57.15,157.48 v59.69,157.48
N$132  (via drill 0.94)
  Bottom 2.032: v49.53,160.02 v52.07,160.02 v54.61,160.02 v57.15,160.02 v59.69,160.02
N$133  (via drill 0.94)
  Bottom 2.032: v49.53,162.56 v52.07,162.56 v54.61,162.56 v57.15,162.56 v59.69,162.56
N$134  (via drill 0.94)
  Bottom 2.032: v49.53,165.1 v52.07,165.1 v54.61,165.1 v57.15,165.1 v59.69,165.1
N$135  (via drill 0.94)
  Bottom 2.032: v49.53,167.64 v52.07,167.64 v54.61,167.64 v57.15,167.64 v59.69,167.64
N$136  (via drill 0.94)
  Bottom 2.032: v49.53,170.18 v52.07,170.18 v54.61,170.18 v57.15,170.18 v59.69,170.18
N$137  (via drill 0.94)
  Bottom 2.032: v49.53,172.72 v52.07,172.72 v54.61,172.72 v57.15,172.72 v59.69,172.72
N$138  (via drill 0.94)
  Bottom 2.032: v49.53,175.26 v52.07,175.26 v54.61,175.26 v57.15,175.26 v59.69,175.26
N$139  (via drill 0.94)
  Bottom 2.032: v49.53,177.8 v52.07,177.8 v54.61,177.8 v57.15,177.8 v59.69,177.8
N$140  (via drill 0.94)
  Bottom 2.032: v49.53,180.34 v52.07,180.34 v54.61,180.34 v57.15,180.34 v59.69,180.34
N$141  (via drill 0.94)
  Bottom 2.032: v49.53,182.88 v52.07,182.88 v54.61,182.88 v57.15,182.88 v59.69,182.88
N$142  (via drill 0.94)
  Bottom 2.032: v49.53,185.42 v52.07,185.42 v54.61,185.42 v57.15,185.42 v59.69,185.42
N$143  (via drill 0.94)
  Bottom 2.032: v49.53,187.96 v52.07,187.96 v54.61,187.96 v57.15,187.96 v59.69,187.96
N$144  (via drill 0.94)
  Bottom 2.032: v49.53,190.5 v52.07,190.5 v54.61,190.5 v57.15,190.5 v59.69,190.5
N$145  (via drill 0.94)
  Bottom 2.032: v49.53,193.04 v52.07,193.04 v54.61,193.04 v57.15,193.04 v59.69,193.04
N$146  (via drill 0.94)
  Bottom 2.032: v49.53,195.58 v52.07,195.58 v54.61,195.58 v57.15,195.58 v59.69,195.58
N$147  (via drill 0.94)
  Bottom 2.032: v49.53,198.12 v52.07,198.12 v54.61,198.12 v57.15,198.12 v59.69,198.12
N$148  (via drill 0.94)
  Bottom 2.032: v49.53,200.66 v52.07,200.66 v54.61,200.66 v57.15,200.66 v59.69,200.66
N$149  (via drill 0.94)
  Bottom 2.032: v49.53,203.2 v52.07,203.2 v54.61,203.2 v57.15,203.2 v59.69,203.2
N$150  (via drill 0.94)
  Bottom 2.032: v49.53,205.74 v52.07,205.74 v54.61,205.74 v57.15,205.74 v59.69,205.74
N$151  (via drill 0.94)
  Bottom 2.032: v49.53,208.28 v52.07,208.28 v54.61,208.28 v57.15,208.28 v59.69,208.28
N$152  (via drill 0.94)
  Bottom 2.032: v49.53,210.82 v52.07,210.82 v54.61,210.82 v57.15,210.82 v59.69,210.82
N$153  (via drill 0.94)
  Bottom 2.032: v49.53,213.36 v52.07,213.36 v54.61,213.36 v57.15,213.36 v59.69,213.36
N$154  (via drill 0.94)
  Bottom 2.032: v49.53,215.9 v52.07,215.9 v54.61,215.9 v57.15,215.9 v59.69,215.9
N$155  (via drill 0.94)
  Bottom 2.032: v49.53,218.44 v52.07,218.44 v54.61,218.44 v57.15,218.44 v59.69,218.44
N$156  (via drill 0.94)
  Bottom 2.032: v49.53,220.98 v52.07,220.98 v54.61,220.98 v57.15,220.98 v59.69,220.98
N$157  (via drill 0.94)
  Bottom 2.032: v49.53,223.52 v52.07,223.52 v54.61,223.52 v57.15,223.52 v59.69,223.52
N$158  (via drill 0.94)
  Bottom 2.032: v49.53,226.06 v52.07,226.06 v54.61,226.06 v57.15,226.06 v59.69,226.06
N$159  (via drill 0.94)
  Bottom 2.032: v49.53,228.6 v52.07,228.6 v54.61,228.6 v57.15,228.6 v59.69,228.6
N$160  (via drill 0.94)
  Bottom 2.032: v49.53,231.14 v52.07,231.14 v54.61,231.14 v57.15,231.14 v59.69,231.14
N$161  (via drill 0.94)
  Bottom 2.032: v49.53,233.68 v52.07,233.68 v54.61,233.68 v57.15,233.68 v59.69,233.68
N$162  (via drill 0.94)
  Bottom 2.032: v49.53,236.22 v52.07,236.22 v54.61,236.22 v57.15,236.22 v59.69,236.22
N$163  (via drill 0.94)
  Bottom 2.032: v49.53,238.76 v52.07,238.76 v54.61,238.76 v57.15,238.76 v59.69,238.76
N$164  (via drill 0.94)
  Bottom 2.032: v49.53,241.3 v52.07,241.3 v54.61,241.3 v57.15,241.3 v59.69,241.3
N$165  (via drill 0.94)
  Bottom 2.032: v49.53,243.84 v52.07,243.84 v54.61,243.84 v57.15,243.84 v59.69,243.84
N$166  (via drill 0.94)
  Bottom 2.032: v49.53,246.38 v52.07,246.38 v54.61,246.38 v57.15,246.38 v59.69,246.38
N$167  (via drill 0.94)
  Bottom 2.032: v49.53,248.92 v52.07,248.92 v54.61,248.92 v57.15,248.92 v59.69,248.92
N$168  (via drill 0.94)
  Bottom 2.032: v49.53,251.46 v52.07,251.46 v54.61,251.46 v57.15,251.46 v59.69,251.46
N$169  (via drill 0.94)
  Bottom 2.032: v49.53,254 v52.07,254 v54.61,254 v57.15,254 v59.69,254
N$170  (via drill 0.94)
  Bottom 2.032: v49.53,256.54 v52.07,256.54 v54.61,256.54 v57.15,256.54 v59.69,256.54
N$171  (via drill 0.94)
  Bottom 2.032: v49.53,259.08 v52.07,259.08 v54.61,259.08 v57.15,259.08 v59.69,259.08
N$172  (via drill 0.94)
  Bottom 2.032: v49.53,261.62 v52.07,261.62 v54.61,261.62 v57.15,261.62 v59.69,261.62
N$173  (via drill 0.94)
  Bottom 2.032: v49.53,264.16 v52.07,264.16 v54.61,264.16 v57.15,264.16 v59.69,264.16
N$174  (via drill 0.94)
  Bottom 2.032: v49.53,266.7 v52.07,266.7 v54.61,266.7 v57.15,266.7 v59.69,266.7
N$175  (via drill 0.94)
  Bottom 2.032: v49.53,269.24 v52.07,269.24 v54.61,269.24 v57.15,269.24 v59.69,269.24
N$176  (via drill 0.94)
  Bottom 2.032: v49.53,271.78 v52.07,271.78 v54.61,271.78 v57.15,271.78 v59.69,271.78
N$177  (via drill 0.94)
  Bottom 2.032: v49.53,274.32 v52.07,274.32 v54.61,274.32 v57.15,274.32 v59.69,274.32
N$178  (via drill 0.94)
  Bottom 2.032: v49.53,276.86 v52.07,276.86 v54.61,276.86 v57.15,276.86 v59.69,276.86
N$179  (via drill 0.94)
  Bottom 2.032: v67.31,12.7 v69.85,12.7 v72.39,12.7 v74.93,12.7 v77.47,12.7
N$180  (via drill 0.94)
  Bottom 2.032: v67.31,15.24 v69.85,15.24 v72.39,15.24 v74.93,15.24 v77.47,15.24
N$181  (via drill 0.94)
  Bottom 2.032: v67.31,17.78 v69.85,17.78 v72.39,17.78 v74.93,17.78 v77.47,17.78
N$182  (via drill 0.94)
  Bottom 2.032: v67.31,20.32 v69.85,20.32 v72.39,20.32 v74.93,20.32 v77.47,20.32
N$183  (via drill 0.94)
  Bottom 2.032: v67.31,22.86 v69.85,22.86 v72.39,22.86 v74.93,22.86 v77.47,22.86
N$184  (via drill 0.94)
  Bottom 2.032: v67.31,25.4 v69.85,25.4 v72.39,25.4 v74.93,25.4 v77.47,25.4
N$185  (via drill 0.94)
  Bottom 2.032: v67.31,27.94 v69.85,27.94 v72.39,27.94 v74.93,27.94 v77.47,27.94
N$186  (via drill 0.94)
  Bottom 2.032: v67.31,30.48 v69.85,30.48 v72.39,30.48 v74.93,30.48 v77.47,30.48
N$187  (via drill 0.94)
  Bottom 2.032: v67.31,33.02 v69.85,33.02 v72.39,33.02 v74.93,33.02 v77.47,33.02
N$188  (via drill 0.94)
  Bottom 2.032: v67.31,35.56 v69.85,35.56 v72.39,35.56 v74.93,35.56 v77.47,35.56
N$189  (via drill 0.94)
  Bottom 2.032: v67.31,38.1 v69.85,38.1 v72.39,38.1 v74.93,38.1 v77.47,38.1
N$190  (via drill 0.94)
  Bottom 2.032: v67.31,40.64 v69.85,40.64 v72.39,40.64 v74.93,40.64 v77.47,40.64
N$191  (via drill 0.94)
  Bottom 2.032: v67.31,43.18 v69.85,43.18 v72.39,43.18 v74.93,43.18 v77.47,43.18
N$192  (via drill 0.94)
  Bottom 2.032: v67.31,45.72 v69.85,45.72 v72.39,45.72 v74.93,45.72 v77.47,45.72
N$193  (via drill 0.94)
  Bottom 2.032: v67.31,48.26 v69.85,48.26 v72.39,48.26 v74.93,48.26 v77.47,48.26
N$194  (via drill 0.94)
  Bottom 2.032: v67.31,50.8 v69.85,50.8 v72.39,50.8 v74.93,50.8 v77.47,50.8
N$195  (via drill 0.94)
  Bottom 2.032: v67.31,53.34 v69.85,53.34 v72.39,53.34 v74.93,53.34 v77.47,53.34
N$196  (via drill 0.94)
  Bottom 2.032: v67.31,55.88 v69.85,55.88 v72.39,55.88 v74.93,55.88 v77.47,55.88
N$197  (via drill 0.94)
  Bottom 2.032: v67.31,58.42 v69.85,58.42 v72.39,58.42 v74.93,58.42 v77.47,58.42
N$198  (via drill 0.94)
  Bottom 2.032: v67.31,60.96 v69.85,60.96 v72.39,60.96 v74.93,60.96 v77.47,60.96
N$199  (via drill 0.94)
  Bottom 2.032: v67.31,63.5 v69.85,63.5 v72.39,63.5 v74.93,63.5 v77.47,63.5
N$200  (via drill 0.94)
  Bottom 2.032: v67.31,66.04 v69.85,66.04 v72.39,66.04 v74.93,66.04 v77.47,66.04
N$201  (via drill 0.94)
  Bottom 2.032: v67.31,68.58 v69.85,68.58 v72.39,68.58 v74.93,68.58 v77.47,68.58
N$202  (via drill 0.94)
  Bottom 2.032: v67.31,71.12 v69.85,71.12 v72.39,71.12 v74.93,71.12 v77.47,71.12
N$203  (via drill 0.94)
  Bottom 2.032: v67.31,73.66 v69.85,73.66 v72.39,73.66 v74.93,73.66 v77.47,73.66
N$204  (via drill 0.94)
  Bottom 2.032: v67.31,76.2 v69.85,76.2 v72.39,76.2 v74.93,76.2 v77.47,76.2
N$205  (via drill 0.94)
  Bottom 2.032: v67.31,78.74 v69.85,78.74 v72.39,78.74 v74.93,78.74 v77.47,78.74
N$206  (via drill 0.94)
  Bottom 2.032: v67.31,81.28 v69.85,81.28 v72.39,81.28 v74.93,81.28 v77.47,81.28
N$207  (via drill 0.94)
  Bottom 2.032: v67.31,83.82 v69.85,83.82 v72.39,83.82 v74.93,83.82 v77.47,83.82
N$208  (via drill 0.94)
  Bottom 2.032: v67.31,86.36 v69.85,86.36 v72.39,86.36 v74.93,86.36 v77.47,86.36
N$209  (via drill 0.94)
  Bottom 2.032: v67.31,88.9 v69.85,88.9 v72.39,88.9 v74.93,88.9 v77.47,88.9
N$210  (via drill 0.94)
  Bottom 2.032: v67.31,91.44 v69.85,91.44 v72.39,91.44 v74.93,91.44 v77.47,91.44
N$211  (via drill 0.94)
  Bottom 2.032: v67.31,93.98 v69.85,93.98 v72.39,93.98 v74.93,93.98 v77.47,93.98
N$212  (via drill 0.94)
  Bottom 2.032: v67.31,96.52 v69.85,96.52 v72.39,96.52 v74.93,96.52 v77.47,96.52
N$213  (via drill 0.94)
  Bottom 2.032: v67.31,99.06 v69.85,99.06 v72.39,99.06 v74.93,99.06 v77.47,99.06
N$214  (via drill 0.94)
  Bottom 2.032: v67.31,101.6 v69.85,101.6 v72.39,101.6 v74.93,101.6 v77.47,101.6
N$215  (via drill 0.94)
  Bottom 2.032: v67.31,104.14 v69.85,104.14 v72.39,104.14 v74.93,104.14 v77.47,104.14
N$216  (via drill 0.94)
  Bottom 2.032: v67.31,106.68 v69.85,106.68 v72.39,106.68 v74.93,106.68 v77.47,106.68
N$217  (via drill 0.94)
  Bottom 2.032: v67.31,109.22 v69.85,109.22 v72.39,109.22 v74.93,109.22 v77.47,109.22
N$218  (via drill 0.94)
  Bottom 2.032: v67.31,111.76 v69.85,111.76 v72.39,111.76 v74.93,111.76 v77.47,111.76
N$219  (via drill 0.94)
  Bottom 2.032: v67.31,114.3 v69.85,114.3 v72.39,114.3 v74.93,114.3 v77.47,114.3
N$220  (via drill 0.94)
  Bottom 2.032: v67.31,116.84 v69.85,116.84 v72.39,116.84 v74.93,116.84 v77.47,116.84
N$221  (via drill 0.94)
  Bottom 2.032: v67.31,119.38 v69.85,119.38 v72.39,119.38 v74.93,119.38 v77.47,119.38
N$222  (via drill 0.94)
  Bottom 2.032: v67.31,121.92 v69.85,121.92 v72.39,121.92 v74.93,121.92 v77.47,121.92
N$223  (via drill 0.94)
  Bottom 2.032: v67.31,124.46 v69.85,124.46 v72.39,124.46 v74.93,124.46 v77.47,124.46
N$224  (via drill 0.94)
  Bottom 2.032: v67.31,127 v69.85,127 v72.39,127 v74.93,127 v77.47,127
N$225  (via drill 0.94)
  Bottom 2.032: v67.31,129.54 v69.85,129.54 v72.39,129.54 v74.93,129.54 v77.47,129.54
N$226  (via drill 0.94)
  Bottom 2.032: v67.31,132.08 v69.85,132.08 v72.39,132.08 v74.93,132.08 v77.47,132.08
N$227  (via drill 0.94)
  Bottom 2.032: v67.31,134.62 v69.85,134.62 v72.39,134.62 v74.93,134.62 v77.47,134.62
N$228  (via drill 0.94)
  Bottom 2.032: v67.31,137.16 v69.85,137.16 v72.39,137.16 v74.93,137.16 v77.47,137.16
N$229  (via drill 0.94)
  Bottom 2.032: v67.31,139.7 v69.85,139.7 v72.39,139.7 v74.93,139.7 v77.47,139.7
N$230  (via drill 0.94)
  Bottom 2.032: v67.31,142.24 v69.85,142.24 v72.39,142.24 v74.93,142.24 v77.47,142.24
N$231  (via drill 0.94)
  Bottom 2.032: v67.31,144.78 v69.85,144.78 v72.39,144.78 v74.93,144.78 v77.47,144.78
N$232  (via drill 0.94)
  Bottom 2.032: v67.31,147.32 v69.85,147.32 v72.39,147.32 v74.93,147.32 v77.47,147.32
N$233  (via drill 0.94)
  Bottom 2.032: v67.31,149.86 v69.85,149.86 v72.39,149.86 v74.93,149.86 v77.47,149.86
N$234  (via drill 0.94)
  Bottom 2.032: v67.31,152.4 v69.85,152.4 v72.39,152.4 v74.93,152.4 v77.47,152.4
N$235  (via drill 0.94)
  Bottom 2.032: v67.31,154.94 v69.85,154.94 v72.39,154.94 v74.93,154.94 v77.47,154.94
N$236  (via drill 0.94)
  Bottom 2.032: v67.31,157.48 v69.85,157.48 v72.39,157.48 v74.93,157.48 v77.47,157.48
N$237  (via drill 0.94)
  Bottom 2.032: v67.31,160.02 v69.85,160.02 v72.39,160.02 v74.93,160.02 v77.47,160.02
N$238  (via drill 0.94)
  Bottom 2.032: v67.31,162.56 v69.85,162.56 v72.39,162.56 v74.93,162.56 v77.47,162.56
N$239  (via drill 0.94)
  Bottom 2.032: v67.31,165.1 v69.85,165.1 v72.39,165.1 v74.93,165.1 v77.47,165.1
N$240  (via drill 0.94)
  Bottom 2.032: v67.31,167.64 v69.85,167.64 v72.39,167.64 v74.93,167.64 v77.47,167.64
N$241  (via drill 0.94)
  Bottom 2.032: v67.31,170.18 v69.85,170.18 v72.39,170.18 v74.93,170.18 v77.47,170.18
N$242  (via drill 0.94)
  Bottom 2.032: v67.31,172.72 v69.85,172.72 v72.39,172.72 v74.93,172.72 v77.47,172.72
N$243  (via drill 0.94)
  Bottom 2.032: v67.31,175.26 v69.85,175.26 v72.39,175.26 v74.93,175.26 v77.47,175.26
N$244  (via drill 0.94)
  Bottom 2.032: v67.31,177.8 v69.85,177.8 v72.39,177.8 v74.93,177.8 v77.47,177.8
N$245  (via drill 0.94)
  Bottom 2.032: v67.31,180.34 v69.85,180.34 v72.39,180.34 v74.93,180.34 v77.47,180.34
N$246  (via drill 0.94)
  Bottom 2.032: v67.31,182.88 v69.85,182.88 v72.39,182.88 v74.93,182.88 v77.47,182.88
N$247  (via drill 0.94)
  Bottom 2.032: v67.31,185.42 v69.85,185.42 v72.39,185.42 v74.93,185.42 v77.47,185.42
N$248  (via drill 0.94)
  Bottom 2.032: v67.31,187.96 v69.85,187.96 v72.39,187.96 v74.93,187.96 v77.47,187.96
N$249  (via drill 0.94)
  Bottom 2.032: v67.31,190.5 v69.85,190.5 v72.39,190.5 v74.93,190.5 v77.47,190.5
N$250  (via drill 0.94)
  Bottom 2.032: v67.31,193.04 v69.85,193.04 v72.39,193.04 v74.93,193.04 v77.47,193.04
N$251  (via drill 0.94)
  Bottom 2.032: v67.31,195.58 v69.85,195.58 v72.39,195.58 v74.93,195.58 v77.47,195.58
N$252  (via drill 0.94)
  Bottom 2.032: v67.31,198.12 v69.85,198.12 v72.39,198.12 v74.93,198.12 v77.47,198.12
N$253  (via drill 0.94)
  Bottom 2.032: v67.31,200.66 v69.85,200.66 v72.39,200.66 v74.93,200.66 v77.47,200.66
N$254  (via drill 0.94)
  Bottom 2.032: v67.31,203.2 v69.85,203.2 v72.39,203.2 v74.93,203.2 v77.47,203.2
N$255  (via drill 0.94)
  Bottom 2.032: v67.31,205.74 v69.85,205.74 v72.39,205.74 v74.93,205.74 v77.47,205.74
N$256  (via drill 0.94)
  Bottom 2.032: v67.31,208.28 v69.85,208.28 v72.39,208.28 v74.93,208.28 v77.47,208.28
N$257  (via drill 0.94)
  Bottom 2.032: v67.31,210.82 v69.85,210.82 v72.39,210.82 v74.93,210.82 v77.47,210.82
N$258  (via drill 0.94)
  Bottom 2.032: v67.31,213.36 v69.85,213.36 v72.39,213.36 v74.93,213.36 v77.47,213.36
N$259  (via drill 0.94)
  Bottom 2.032: v67.31,215.9 v69.85,215.9 v72.39,215.9 v74.93,215.9 v77.47,215.9
N$260  (via drill 0.94)
  Bottom 2.032: v67.31,218.44 v69.85,218.44 v72.39,218.44 v74.93,218.44 v77.47,218.44
N$261  (via drill 0.94)
  Bottom 2.032: v67.31,220.98 v69.85,220.98 v72.39,220.98 v74.93,220.98 v77.47,220.98
N$262  (via drill 0.94)
  Bottom 2.032: v67.31,223.52 v69.85,223.52 v72.39,223.52 v74.93,223.52 v77.47,223.52
N$263  (via drill 0.94)
  Bottom 2.032: v67.31,226.06 v69.85,226.06 v72.39,226.06 v74.93,226.06 v77.47,226.06
N$264  (via drill 0.94)
  Bottom 2.032: v67.31,228.6 v69.85,228.6 v72.39,228.6 v74.93,228.6 v77.47,228.6
N$265  (via drill 0.94)
  Bottom 2.032: v67.31,231.14 v69.85,231.14 v72.39,231.14 v74.93,231.14 v77.47,231.14
N$266  (via drill 0.94)
  Bottom 2.032: v67.31,233.68 v69.85,233.68 v72.39,233.68 v74.93,233.68 v77.47,233.68
N$267  (via drill 0.94)
  Bottom 2.032: v67.31,236.22 v69.85,236.22 v72.39,236.22 v74.93,236.22 v77.47,236.22
N$268  (via drill 0.94)
  Bottom 2.032: v67.31,238.76 v69.85,238.76 v72.39,238.76 v74.93,238.76 v77.47,238.76
N$269  (via drill 0.94)
  Bottom 2.032: v67.31,241.3 v69.85,241.3 v72.39,241.3 v74.93,241.3 v77.47,241.3
N$270  (via drill 0.94)
  Bottom 2.032: v67.31,243.84 v69.85,243.84 v72.39,243.84 v74.93,243.84 v77.47,243.84
N$271  (via drill 0.94)
  Bottom 2.032: v67.31,246.38 v69.85,246.38 v72.39,246.38 v74.93,246.38 v77.47,246.38
N$272  (via drill 0.94)
  Bottom 2.032: v67.31,248.92 v69.85,248.92 v72.39,248.92 v74.93,248.92 v77.47,248.92
N$273  (via drill 0.94)
  Bottom 2.032: v67.31,251.46 v69.85,251.46 v72.39,251.46 v74.93,251.46 v77.47,251.46
N$274  (via drill 0.94)
  Bottom 2.032: v67.31,254 v69.85,254 v72.39,254 v74.93,254 v77.47,254
N$275  (via drill 0.94)
  Bottom 2.032: v67.31,256.54 v69.85,256.54 v72.39,256.54 v74.93,256.54 v77.47,256.54
N$276  (via drill 0.94)
  Bottom 2.032: v67.31,259.08 v69.85,259.08 v72.39,259.08 v74.93,259.08 v77.47,259.08
N$277  (via drill 0.94)
  Bottom 2.032: v67.31,261.62 v69.85,261.62 v72.39,261.62 v74.93,261.62 v77.47,261.62
N$278  (via drill 0.94)
  Bottom 2.032: v67.31,264.16 v69.85,264.16 v72.39,264.16 v74.93,264.16 v77.47,264.16
N$279  (via drill 0.94)
  Bottom 2.032: v67.31,266.7 v69.85,266.7 v72.39,266.7 v74.93,266.7 v77.47,266.7
N$280  (via drill 0.94)
  Bottom 2.032: v67.31,269.24 v69.85,269.24 v72.39,269.24 v74.93,269.24 v77.47,269.24
N$281  (via drill 0.94)
  Bottom 2.032: v67.31,271.78 v69.85,271.78 v72.39,271.78 v74.93,271.78 v77.47,271.78
N$282  (via drill 0.94)
  Bottom 2.032: v67.31,274.32 v69.85,274.32 v72.39,274.32 v74.93,274.32 v77.47,274.32
N$283  (via drill 0.94)
  Bottom 2.032: v67.31,276.86 v69.85,276.86 v72.39,276.86 v74.93,276.86 v77.47,276.86
N$284  (via drill 0.94)
  Bottom 2.032: v80.01,12.7 v82.55,12.7 v85.09,12.7 v87.63,12.7 v90.17,12.7
N$285  (via drill 0.94)
  Bottom 2.032: v80.01,15.24 v82.55,15.24 v85.09,15.24 v87.63,15.24 v90.17,15.24
N$286  (via drill 0.94)
  Bottom 2.032: v80.01,17.78 v82.55,17.78 v85.09,17.78 v87.63,17.78 v90.17,17.78
N$287  (via drill 0.94)
  Bottom 2.032: v80.01,20.32 v82.55,20.32 v85.09,20.32 v87.63,20.32 v90.17,20.32
N$288  (via drill 0.94)
  Bottom 2.032: v80.01,22.86 v82.55,22.86 v85.09,22.86 v87.63,22.86 v90.17,22.86
N$289  (via drill 0.94)
  Bottom 2.032: v80.01,25.4 v82.55,25.4 v85.09,25.4 v87.63,25.4 v90.17,25.4
N$290  (via drill 0.94)
  Bottom 2.032: v80.01,27.94 v82.55,27.94 v85.09,27.94 v87.63,27.94 v90.17,27.94
N$291  (via drill 0.94)
  Bottom 2.032: v80.01,30.48 v82.55,30.48 v85.09,30.48 v87.63,30.48 v90.17,30.48
N$292  (via drill 0.94)
  Bottom 2.032: v80.01,33.02 v82.55,33.02 v85.09,33.02 v87.63,33.02 v90.17,33.02
N$293  (via drill 0.94)
  Bottom 2.032: v80.01,35.56 v82.55,35.56 v85.09,35.56 v87.63,35.56 v90.17,35.56
N$294  (via drill 0.94)
  Bottom 2.032: v80.01,38.1 v82.55,38.1 v85.09,38.1 v87.63,38.1 v90.17,38.1
N$295  (via drill 0.94)
  Bottom 2.032: v80.01,40.64 v82.55,40.64 v85.09,40.64 v87.63,40.64 v90.17,40.64
N$296  (via drill 0.94)
  Bottom 2.032: v80.01,43.18 v82.55,43.18 v85.09,43.18 v87.63,43.18 v90.17,43.18
N$297  (via drill 0.94)
  Bottom 2.032: v80.01,45.72 v82.55,45.72 v85.09,45.72 v87.63,45.72 v90.17,45.72
N$298  (via drill 0.94)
